FUNCTION_BLOCK IC_KP2_2HB21_IUH_MF
VAR_INPUT
	pADR_IN:								PVOID;					(* Pointer array input data *)
	cbSIZE_IN:								UDINT;					(* Size array input data *)
	pADR_OUT:								PVOID;					(* Pointer array output data *)
	cbSIZE_OUT:								UDINT;					(* Size array output data *)	
	I_T_Timeout : 							TIME;					// Timeout to check command responses
	I_b_StartRead : 						BOOL;					// Trigger to start read command
	I_b_StartWrite : 						BOOL;					// Trigger to start write command
	I_b_StartSpecialCommand : 				BOOL;					// Trigger to start special command (user defined command)
	I_b_UserMemory_UID : 					BOOL;					//0 := access to User Memory; 1 := access to UID/Fixcode
	I_b_EPC : 								BOOL;					//0 := configuration done by Head1UserMemoryUID active; 1 := access to UII/EPC Code (UHF only)
	I_b_SingleEnhanced : 					BOOL;					// 0 = Single command (one-time) ; 1 = Enhanced command (permanent)
	I_b_Quit : 								BOOL;					// Trigger to start Quit command (abort Enhanced command)
	I_w_StartAddress : 						WORD;					// Startaddress of memory access 
	I_i_WordNumber : 						INT;					// Number of blocks
	I_w_TagType : 							WORD;					// TagType
	I_b_WriteParameter : 					BOOL;					//0 := read access to parameter; 1 := write access to parameter
END_VAR
VAR_OUTPUT
	O_b_Done : 								BOOL;					//0 = tag leave detection zone (Enhanced); 1 = tag access successfully executed
	O_b_NoDataCarrier : 					BOOL;					//0 = tag inside/enter detection zone; 1 = no tag or tag leave detection zone
	O_b_Busy : 								BOOL;					//0 = no command actiive; 1 = command active
	O_b_Finish : 							BOOL;					//0 = command active; 1 = command finished
	O_b_Error : 							BOOL;					//0 = no error state; 1 = error state active; check status value
	O_B_Status : 							BYTE;					//Status value of the command response; error information
	O_B_ReplyCounter : 						BYTE;					//Counter of the command responses; increment each new response
	O_b_EndConfig : 						BOOL;					//1 = parameter access finished
END_VAR
VAR_IN_OUT
	IO_b_SetRestart : 						BOOL;					//Trigger initialisation routine
	IO_b_InitFinish : 						BOOL;					//Initialisation routine finished
	IO_b_NewData :							BOOL;					//1 = new data inside data block aviable; direct reset by the user neccessary
	IO_b_StartConfig : 						BOOL;					//1 = trigger of parameter access
	UserDataGlobal 	: 						IDENTControl_UserData_IUH_MF;	//Data block for read/write data and parameter data
END_VAR
VAR
	IDENTControl_FB_MF		: 				IDENTControl_MF;		//Definition of internal function block for Single Frame Protocol
	SpecialCommand_Internal: 				BOOL;					//internal signal for trigger of Special command
	ConfigActive : 							BOOL;					//execution of Special command active
	StateConfig : 							INT;					//state of the execution list
	Done_Internal : 						BOOL;					//Special command finished
	i : 									INT := 0;				//counter
END_VAR

	(*
	#############################################################################################
	
	General Header
	------------------------------------------------------------------------------------------
	Short description:  Function Block for IC-KP2-2HB21 MultiFrame with Parameter configuration for IUH-F19x-V1-FRx-XX
	Version:            1.0
	Name:               IC-KP2-2HB21 Multiframe Protocol with UHF Parameter configuration for IUH-F19x-V1-FRx-XX
	Date:               2024-11-13
	Company:            Pepperl+Fuchs SE
	Author:             Karsten Reinhardt
	EMail:              kreinhardt@de.pepperl-fuchs.com
	Phone:              +49 (0) 621 776 1736

	Changes 1.0: first release
	    - function block include a further function block for standard read/write command without automatic parameter
	    configuration;    
	    - read and write access for different UHF parameter
	
	------------------------------------------------------------------------------------------
	    
	#############################################################################################
	*)

	(*input SpecialCommand hand over to internal signal*)
	SpecialCommand_Internal                   			:= I_b_StartSpecialCommand;

	(*Increase the state of the configuration counter*)
	IF ConfigActive = TRUE AND O_b_Done = TRUE THEN
	    ConfigActive                         			:= FALSE;
	    StateConfig                          			:= StateConfig + 1;
	END_IF;
	
	(*Set Status of the configuration counter to 1 with the trigger for the start of the configuration*)
	IF IO_b_StartConfig = TRUE THEN
	    StateConfig                          			:= 1;
	    IO_b_StartConfig                          		:= FALSE;
	    O_b_EndConfig                             		:= FALSE;
	END_IF;

	IF NOT ConfigActive THEN
	    CASE StateConfig OF
	            
	        0: (* ***** Idle state ***** *)
	            ;
	            
	        1:  (*Additional Information - Parameter IF; transmit a further information telegram with RSSI value;
	            if this parameter is activated a further status 16#0B telegram will transmitted by the evaluation
	            unit; this telegram follows directly after the status 16#00 telegram which contains the read in data
	            of a tag; the status 16#0B telegram with the information will send only one time after the tag is detected;
	            in default setting the parameter is switched off and no additional information are transmit*)
	            IF I_b_WriteParameter = TRUE THEN
	                UserDataGlobal.SpecialCommand[0] 	:= 16#BF;
	            ELSE
					UserDataGlobal.SpecialCommand[0] 	:= 16#BE;	                
	            END_IF;
	            UserDataGlobal.SpecialCommand[1]        := 16#00;
	            UserDataGlobal.SpecialCommand[2]        := 16#00;
	            UserDataGlobal.SpecialCommand[3]        := 16#55;      //SystemCode U
	            UserDataGlobal.SpecialCommand[4]        := 16#49;      //Parameter sign High Byte 'I'
	            UserDataGlobal.SpecialCommand[5]        := 16#46;      //Parameter sign Low Byte 'F'
				IF I_b_WriteParameter = TRUE THEN
	                UserDataGlobal.SpecialCommand[6]    := 16#00;    //Length Parameter High Byte 
	                UserDataGlobal.SpecialCommand[7]    := 16#01;    //Length Parameter Low Byte 
	                UserDataGlobal.SpecialCommand[8]    := UserDataGlobal.WriteParam_IF;    //Parameter value; 16#00 Switched off; 16#01 Switched on
	            ELSE
	                UserDataGlobal.SpecialCommand[6]    := 16#00;    //Length Parameter High Byte 
	                UserDataGlobal.SpecialCommand[7]    := 16#00;    //Length Parameter Low Byte 
	                UserDataGlobal.SpecialCommand[8]    := 16#00;
	            END_IF;
	            SpecialCommand_Internal       			:= TRUE;
	            ConfigActive                 			:= TRUE;            
				
	        2:  (*Antenna Polarisation - Parameter AP; change the polarisation plane of the antenna;
            	in default setting the combined mode is activated. In this case the antenna executes an invetury
            	in horizontal and vertical polarisation plane; this has the advantage that the orientation of the
            	tag can different; of the tag orientation is always identical it is possible to switch to horizontal
            	or vertical polarisation plane; this reduce the execution time for a command*)
	            IF I_b_WriteParameter = TRUE THEN
	                UserDataGlobal.SpecialCommand[0]    := 16#BF;
	            ELSE
	                UserDataGlobal.SpecialCommand[0]    := 16#BE;
	            END_IF;
	            UserDataGlobal.SpecialCommand[1]        := 16#00;
	            UserDataGlobal.SpecialCommand[2]        := 16#00;
	            UserDataGlobal.SpecialCommand[3]        := 16#55;      //SystemCode U
	            UserDataGlobal.SpecialCommand[4]        := 16#41;      //Parameter sign High Byte 'A'
	            UserDataGlobal.SpecialCommand[5]        := 16#50;      //Parameter sign Low Byte 'P'
	            IF I_b_WriteParameter = TRUE THEN
	                UserDataGlobal.SpecialCommand[6]    := 16#00;    //Length Parameter High Byte 
	                UserDataGlobal.SpecialCommand[7]    := 16#01;    //Length Parameter Low Byte 
	                UserDataGlobal.SpecialCommand[8]    := UserDataGlobal.WriteParam_AP;    //Parameter value; 16#43 = Combined Mode; 16#48 = horizontal; 16#56 = vertical
	            ELSE
	                UserDataGlobal.SpecialCommand[6]    := 16#00;    //Length Parameter High Byte 
	                UserDataGlobal.SpecialCommand[7]    := 16#00;    //Length Parameter Low Byte 
	                UserDataGlobal.SpecialCommand[8]    := 16#00;    //Parameter value; 
	            END_IF;
	            SpecialCommand_Internal       			:= TRUE;
	            ConfigActive 							:= TRUE;

	        3:  (*Sending Channels - Parameter CD; used channels on the air interface
            	the FR1-01 devce version uses up to 4 channels on the air interface; with this parameter you can reduce
            	the number of the channels and also define the order of the channels; by reducing the number of channels
            	you achieve a reduction of the execution time; if severla readers are close to each other you can define
            	different air interface channels for the reader to avoid influences*)
	            IF I_b_WriteParameter = TRUE THEN
	                UserDataGlobal.SpecialCommand[0]    := 16#BF;
	            ELSE
	                UserDataGlobal.SpecialCommand[0]    := 16#BE;
	            END_IF;
	            UserDataGlobal.SpecialCommand[1]        := 16#00;
	            UserDataGlobal.SpecialCommand[2]        := 16#00;
	            UserDataGlobal.SpecialCommand[3]        := 16#55;      //SystemCode U
	            UserDataGlobal.SpecialCommand[4]        := 16#43;      //Parameter sign High Byte 'C'
	            UserDataGlobal.SpecialCommand[5]        := 16#44;      //Parameter sign Low Byte 'D'
	            IF I_b_WriteParameter = TRUE THEN
	                UserDataGlobal.SpecialCommand[6]    := INT_TO_BYTE (SHR (UserDataGlobal.Length_CD, 8));    //Length Parameter High Byte 
	                UserDataGlobal.SpecialCommand[7]    := INT_TO_BYTE (UserDataGlobal.Length_CD);    //Length Parameter Low Byte
	                UserDataGlobal.SpecialCommand[8]    := UserDataGlobal.WriteParam_CD[0];    //Parameter value; value Parameter CD
	                UserDataGlobal.SpecialCommand[9]    := UserDataGlobal.WriteParam_CD[1];    //Parameter value; value Parameter CD
	                UserDataGlobal.SpecialCommand[10]   := UserDataGlobal.WriteParam_CD[2];    //Parameter value; value Parameter CD
	                UserDataGlobal.SpecialCommand[11]   := UserDataGlobal.WriteParam_CD[3];    //Parameter value; value Parameter CD
	            ELSE
	                UserDataGlobal.SpecialCommand[6]    := 16#00;    //Length Parameter High Byte 
	                UserDataGlobal.SpecialCommand[7]    := 16#00;    //Length Parameter Low Byte 
	                UserDataGlobal.SpecialCommand[8]    := 16#00;    //Parameter value; 
	                UserDataGlobal.SpecialCommand[9]    := 16#00;    //Parameter value; 
	                UserDataGlobal.SpecialCommand[10]   := 16#00;    //Parameter value; 
	                UserDataGlobal.SpecialCommand[11]   := 16#00;    //Parameter value; 
	            END_IF;
	            SpecialCommand_Internal       			:= TRUE;
	            ConfigActive                 			:= TRUE;			
				
 			4:  (*Enhanced Status 5 - Parameter E5; delay the sending of a status 16#05 telegram which signalise that
            	a tag leaves the detection zone; if there is a inhomogeneous reading zone you have areas in which a tag
           		could not identified; in this case the reader generates a status 16#05 telegram that signalize that a tag 
            	could not accessed; these parameter can delay such telegrams that you can avoid a lot of status 16#05 (no read) 
            	telegrams in a inhomogeneous reading zone*)
	            IF I_b_WriteParameter = TRUE THEN
	                UserDataGlobal.SpecialCommand[0]    := 16#BF;
	            ELSE
	                UserDataGlobal.SpecialCommand[0]    := 16#BE;
	            END_IF;
	            UserDataGlobal.SpecialCommand[1]        := 16#00;
	            UserDataGlobal.SpecialCommand[2]        := 16#00;
	            UserDataGlobal.SpecialCommand[3]        := 16#55;      //SystemCode U
	            UserDataGlobal.SpecialCommand[4]        := 16#45;      //Parameter sign High Byte 'E'
	            UserDataGlobal.SpecialCommand[5]        := 16#35;      //Parameter sign Low Byte '5'
	            IF I_b_WriteParameter = TRUE THEN
	                UserDataGlobal.SpecialCommand[6]    := 16#00;    //Length Parameter High Byte 
	                UserDataGlobal.SpecialCommand[7]    := 16#01;    //Length Parameter Low Byte 
	                UserDataGlobal.SpecialCommand[8]    := UserDataGlobal.WriteParam_E5;    //Parameter value; 16#05 = Default setting
	            ELSE
	                UserDataGlobal.SpecialCommand[6]    := 16#00;    //Length Parameter High Byte 
	                UserDataGlobal.SpecialCommand[7]    := 16#00;    //Length Parameter Low Byte 
	                UserDataGlobal.SpecialCommand[8]    := 16#00;    //Parameter value;
	            END_IF;
	            SpecialCommand_Internal       			:= TRUE;
	            ConfigActive                 			:= TRUE;			
				
	        5: (*Memory Bank - Parameter MB; define to which memory bank the Single/Enhanced Read/Write Words commands
            	get access; in default setting the Read/Write Words command get access to memory bank 16#03 "User Memory";
            	16#00 --> Password Area; 16#01 --> UII/EPC; 16#02 --> TID; 16#03 --> User Memory*)
	            IF I_b_WriteParameter = TRUE THEN
	                UserDataGlobal.SpecialCommand[0]    := 16#BF;
	            ELSE
	                UserDataGlobal.SpecialCommand[0]    := 16#BE;
	            END_IF;
	            UserDataGlobal.SpecialCommand[1]        := 16#00;
	            UserDataGlobal.SpecialCommand[2]        := 16#00;
	            UserDataGlobal.SpecialCommand[3]        := 16#55;      //SystemCode U
	            UserDataGlobal.SpecialCommand[4]        := 16#4D;      //Parameter sign High Byte 'M'
	            UserDataGlobal.SpecialCommand[5]        := 16#42;      //Parameter sign Low Byte 'B'
	            IF I_b_WriteParameter = TRUE THEN
	                UserDataGlobal.SpecialCommand[6]    := 16#00;    //Length Parameter High Byte 
	                UserDataGlobal.SpecialCommand[7]    := 16#01;    //Length Parameter Low Byte 
	                UserDataGlobal.SpecialCommand[8]    := UserDataGlobal.WriteParam_MB;    //Parameter value; Default = 16#03 = User Memory
	            ELSE
	                UserDataGlobal.SpecialCommand[6]    := 16#00;    //Length Parameter High Byte 
	                UserDataGlobal.SpecialCommand[7]    := 16#00;    //Length Parameter Low Byte 
	                UserDataGlobal.SpecialCommand[8]    := 16#00;    //Parameter value; 
	            END_IF;
	            SpecialCommand_Internal       			:= TRUE;
	            ConfigActive                 			:= TRUE;	            	
				
	        6:  (*Number of Tags - Parameter NT; stop criteria to abort the execution of a Single command; this parameter
            	allows the stop of the command execution if one or a defined number of tags are detected; in default setting
            	the parameter has the value 16#FF and the command does not stop before all invetury rounds are executed; if
            	the value 16#01 is defined the command execution of a Single command stops if one tag is detected during an
            	invetury round; if two tags are detected during an inventury round both tags will transmit*)
	            IF I_b_WriteParameter = TRUE THEN
	                UserDataGlobal.SpecialCommand[0]    := 16#BF;
	            ELSE
	                UserDataGlobal.SpecialCommand[0]    := 16#BE;
	            END_IF;
	            UserDataGlobal.SpecialCommand[1]        := 16#00;
	            UserDataGlobal.SpecialCommand[2]        := 16#00;
	            UserDataGlobal.SpecialCommand[3]        := 16#55;      //SystemCode U
	            UserDataGlobal.SpecialCommand[4]        := 16#4E;      //Parameter sign High Byte 'N'
	            UserDataGlobal.SpecialCommand[5]        := 16#54;      //Parameter sign Low Byte 'T'
	            IF I_b_WriteParameter = TRUE THEN
	                UserDataGlobal.SpecialCommand[6]    := 16#00;    //Length Parameter High Byte 
	                UserDataGlobal.SpecialCommand[7]    := 16#01;    //Length Parameter Low Byte 
	                UserDataGlobal.SpecialCommand[8]    := UserDataGlobal.WriteParam_NT;    //Parameter value; Default = 16#FF
	            ELSE
	                UserDataGlobal.SpecialCommand[6]    := 16#00;    //Length Parameter High Byte 
	                UserDataGlobal.SpecialCommand[7]    := 16#00;    //Length Parameter Low Byte 
	                UserDataGlobal.SpecialCommand[8]    := 16#00;    //Parameter value; 
	            END_IF;
	            SpecialCommand_Internal       			:= TRUE;
	            ConfigActive                 			:= TRUE;
	            
	        7:  (*Protocol Mode - Parameter QV; defines the communication protocol of the head; in default setting the
            	head communicates with the MultiFrame protocol; this allows the identification of several tags inside
            	the detection zone; it is possible to switch the protocol to SingleFrame, but than the function block
            	is incompatible*)
	            IF I_b_WriteParameter = TRUE THEN
	                UserDataGlobal.SpecialCommand[0]    := 16#BF;
	            ELSE
	                UserDataGlobal.SpecialCommand[0]    := 16#BE;
	            END_IF;
	            UserDataGlobal.SpecialCommand[1]        := 16#00;
	            UserDataGlobal.SpecialCommand[2]        := 16#00;
	            UserDataGlobal.SpecialCommand[3]        := 16#55;      //SystemCode U
	            UserDataGlobal.SpecialCommand[4]        := 16#51;      //Parameter sign High Byte 'Q'
	            UserDataGlobal.SpecialCommand[5]        := 16#56;      //Parameter sign Low Byte 'V'
	            IF I_b_WriteParameter = TRUE THEN
	                UserDataGlobal.SpecialCommand[6]    := 16#00;    //Length Parameter High Byte 
	                UserDataGlobal.SpecialCommand[7]    := 16#01;    //Length Parameter Low Byte 
	                UserDataGlobal.SpecialCommand[8]    := UserDataGlobal.WriteParam_QV;    //Parameter value; 
	            ELSE
	                UserDataGlobal.SpecialCommand[6]    := 16#00;    //Length Parameter High Byte 
	                UserDataGlobal.SpecialCommand[7]    := 16#00;    //Length Parameter Low Byte 
	                UserDataGlobal.SpecialCommand[8]    := 16#00;    //Parameter value; 
	            END_IF;
	            SpecialCommand_Internal       			:= TRUE;
	            ConfigActive                 			:= TRUE;								

			8:  (*Q Value - Parameter QW; defines the number of time slots on the air interface with 2^Q; the number of
            	time slots should be fit to the number of tags which should be identified*)
	            IF I_b_WriteParameter = TRUE THEN
	                UserDataGlobal.SpecialCommand[0]    := 16#BF;
	            ELSE
	                UserDataGlobal.SpecialCommand[0]    := 16#BE;
	            END_IF;
	            UserDataGlobal.SpecialCommand[1]        := 16#00;
	            UserDataGlobal.SpecialCommand[2]        := 16#00;
	            UserDataGlobal.SpecialCommand[3]        := 16#55;      //SystemCode U
	            UserDataGlobal.SpecialCommand[4]        := 16#51;      //Parameter sign High Byte 'Q'
	            UserDataGlobal.SpecialCommand[5]        := 16#57;      //Parameter sign Low Byte 'W'
	            IF I_b_WriteParameter = TRUE THEN
	                UserDataGlobal.SpecialCommand[6]    := 16#00;    //Length Parameter High Byte 
	                UserDataGlobal.SpecialCommand[7]    := 16#01;    //Length Parameter Low Byte 
	                UserDataGlobal.SpecialCommand[8]    := UserDataGlobal.WriteParam_QW;
	                UserDataGlobal.SpecialCommand[9]    := 16#00;
	            ELSE
	                UserDataGlobal.SpecialCommand[6]    := 16#00;    //Length Parameter High Byte 
	                UserDataGlobal.SpecialCommand[7]    := 16#00;    //Length Parameter Low Byte 
	                UserDataGlobal.SpecialCommand[8]    := 16#00;    //Parameter value; 
	                UserDataGlobal.SpecialCommand[9]    := 16#00;    //Parameter value; 
	            END_IF;
	            SpecialCommand_Internal       			:= TRUE;
	            ConfigActive                 			:= TRUE;	
								
			9:  (*Sensing Mode - Parameter SM; defines a pause time during the execution of Enhanced commands; by increasing
            	the pause time it is possible to reduce the internal heating of the head *)
	            IF I_b_WriteParameter = TRUE THEN
	                UserDataGlobal.SpecialCommand[0]    := 16#BF;
	            ELSE
	                UserDataGlobal.SpecialCommand[0]    := 16#BE;
	            END_IF;
	            UserDataGlobal.SpecialCommand[1]        := 16#00;
	            UserDataGlobal.SpecialCommand[2]        := 16#00;
	            UserDataGlobal.SpecialCommand[3]        := 16#55;      //SystemCode U
	            UserDataGlobal.SpecialCommand[4]        := 16#53;      //Parameter sign High Byte 'S'
	            UserDataGlobal.SpecialCommand[5]        := 16#4D;      //Parameter sign Low Byte 'M'
	            IF I_b_WriteParameter = TRUE THEN
	                UserDataGlobal.SpecialCommand[6]    := 16#00;    //Length Parameter High Byte 
	                UserDataGlobal.SpecialCommand[7]    := 16#02;    //Length Parameter Low Byte 
	                UserDataGlobal.SpecialCommand[8]    := WORD_TO_BYTE (SHR (UserDataGlobal.WriteParam_SM, 8));
					UserDataGlobal.SpecialCommand[9]    := WORD_TO_BYTE (UserDataGlobal.WriteParam_SM);    //Parameter value; 
	            ELSE
	                UserDataGlobal.SpecialCommand[6]    := 16#00;    //Length Parameter High Byte 
	                UserDataGlobal.SpecialCommand[7]    := 16#00;    //Length Parameter Low Byte 
	                UserDataGlobal.SpecialCommand[8]    := 16#00;    //Parameter value; 
	                UserDataGlobal.SpecialCommand[9]    := 16#00;    //Parameter value; 
	            END_IF;
	            SpecialCommand_Internal       			:= TRUE;
	            ConfigActive                 			:= TRUE;							
				
	        10:  (*Tries allowed - Parameter TA; defines the number of allowed tries for the identification of a tag*)
	            IF I_b_WriteParameter = TRUE THEN
	                UserDataGlobal.SpecialCommand[0]    := 16#BF;
	            ELSE
	                UserDataGlobal.SpecialCommand[0]    := 16#BE;
	            END_IF;
	            UserDataGlobal.SpecialCommand[1]        := 16#00;
	            UserDataGlobal.SpecialCommand[2]        := 16#00;
	            UserDataGlobal.SpecialCommand[3]        := 16#55;      //SystemCode U
	            UserDataGlobal.SpecialCommand[4]        := 16#54;      //Parameter sign High Byte 'T'
	            UserDataGlobal.SpecialCommand[5]        := 16#41;      //Parameter sign Low Byte 'A'
	            IF I_b_WriteParameter = TRUE THEN
	                UserDataGlobal.SpecialCommand[6]    := 16#00;    //Length Parameter High Byte 
	                UserDataGlobal.SpecialCommand[7]    := 16#01;    //Length Parameter Low Byte 
	                UserDataGlobal.SpecialCommand[8]    := UserDataGlobal.WriteParam_TA;
	                UserDataGlobal.SpecialCommand[9]    := 16#00;	           
 				ELSE
	                UserDataGlobal.SpecialCommand[6]    := 16#00;    //Length Parameter High Byte 
	                UserDataGlobal.SpecialCommand[7]    := 16#00;    //Length Parameter Low Byte 
	                UserDataGlobal.SpecialCommand[8]    := 16#00;    //Parameter value; 
	            END_IF;
	            SpecialCommand_Internal       			:= TRUE;
	            ConfigActive                 			:= TRUE;				
												
	        11:  (*Power Transmit - Parameter PT; defines the output power of the RFID antenna; it is allowed to define up
            	10 different levels for this parameter; in this case it is possible to generate a ramp for the output power;
           		following levels are possible (in mW) 3, 4, 5, 6, 8, 10, 13, 15, 20, 25, 30, 40, 50, 60, 80, 100, 125, 150,
            	200, 250, 300, 400, 500, 600, 800, 1000, 1250, 1500, 2000*)
	            IF I_b_WriteParameter = TRUE THEN
	                UserDataGlobal.SpecialCommand[0]    := 16#BF;
	            ELSE
	                UserDataGlobal.SpecialCommand[0]    := 16#BE;
	            END_IF;
	            UserDataGlobal.SpecialCommand[1]        := 16#00;
	            UserDataGlobal.SpecialCommand[2]        := 16#00;
	            UserDataGlobal.SpecialCommand[3]        := 16#55;      //SystemCode U
	            UserDataGlobal.SpecialCommand[4]        := 16#50;      //Parameter sign High Byte 'P'
	            UserDataGlobal.SpecialCommand[5]        := 16#54;      //Parameter sign Low Byte 'T'
	            IF I_b_WriteParameter = TRUE THEN
	                UserDataGlobal.SpecialCommand[6]    := INT_TO_BYTE (SHR (UserDataGlobal.Length_PT, 8));    //Length Parameter High Byte 
	                UserDataGlobal.SpecialCommand[7]    := INT_TO_BYTE (UserDataGlobal.Length_PT);    //Length Parameter Low Byte 
	            	UserDataGlobal.SpecialCommand[8]    := WORD_TO_BYTE (SHR (UserDataGlobal.WriteParam_PT[1], 8));
					UserDataGlobal.SpecialCommand[9]	:= WORD_TO_BYTE (UserDataGlobal.WriteParam_PT[1]);
					UserDataGlobal.SpecialCommand[10]   := WORD_TO_BYTE (SHR (UserDataGlobal.WriteParam_PT[2], 8));
					UserDataGlobal.SpecialCommand[11]	:= WORD_TO_BYTE (UserDataGlobal.WriteParam_PT[2]);
					UserDataGlobal.SpecialCommand[12]   := WORD_TO_BYTE (SHR (UserDataGlobal.WriteParam_PT[3], 8));
					UserDataGlobal.SpecialCommand[13]	:= WORD_TO_BYTE (UserDataGlobal.WriteParam_PT[3]);
					UserDataGlobal.SpecialCommand[14]   := WORD_TO_BYTE (SHR (UserDataGlobal.WriteParam_PT[4], 8));
					UserDataGlobal.SpecialCommand[15]	:= WORD_TO_BYTE (UserDataGlobal.WriteParam_PT[4]);
					UserDataGlobal.SpecialCommand[16]   := WORD_TO_BYTE (SHR (UserDataGlobal.WriteParam_PT[5], 8));
					UserDataGlobal.SpecialCommand[17]	:= WORD_TO_BYTE (UserDataGlobal.WriteParam_PT[5]);
					UserDataGlobal.SpecialCommand[18]   := WORD_TO_BYTE (SHR (UserDataGlobal.WriteParam_PT[6], 8));
					UserDataGlobal.SpecialCommand[19]	:= WORD_TO_BYTE (UserDataGlobal.WriteParam_PT[6]);
					UserDataGlobal.SpecialCommand[20]   := WORD_TO_BYTE (SHR (UserDataGlobal.WriteParam_PT[7], 8));
					UserDataGlobal.SpecialCommand[21]	:= WORD_TO_BYTE (UserDataGlobal.WriteParam_PT[7]);
					UserDataGlobal.SpecialCommand[22]   := WORD_TO_BYTE (SHR (UserDataGlobal.WriteParam_PT[8], 8));
					UserDataGlobal.SpecialCommand[23]	:= WORD_TO_BYTE (UserDataGlobal.WriteParam_PT[8]);
					UserDataGlobal.SpecialCommand[24]   := WORD_TO_BYTE (SHR (UserDataGlobal.WriteParam_PT[9], 8));
					UserDataGlobal.SpecialCommand[25]	:= WORD_TO_BYTE (UserDataGlobal.WriteParam_PT[9]);
					UserDataGlobal.SpecialCommand[26]   := WORD_TO_BYTE (SHR (UserDataGlobal.WriteParam_PT[10], 8));
					UserDataGlobal.SpecialCommand[27]	:= WORD_TO_BYTE (UserDataGlobal.WriteParam_PT[10]);
				ELSE
	                UserDataGlobal.SpecialCommand[6]    := 16#00;    //Length Parameter High Byte 
	                UserDataGlobal.SpecialCommand[7]    := 16#00;    //Length Parameter Low Byte 
	                UserDataGlobal.SpecialCommand[8]    := 16#00;    //Parameter value; 
	                UserDataGlobal.SpecialCommand[9]    := 16#00;    //Parameter value; 
	            END_IF;
	            SpecialCommand_Internal 				:= TRUE;
	            ConfigActive 							:= TRUE;
		
				
	        12:    (*Measured Reflection - Parameter MF; read out measured reflection; the measurement of the reflection
                is only possible if the antenna polarisation is horizontal (H) or vertical (V); in default setting
                the parameter AP "antenna polarisation" is defined as "C" combined; in this case the measurement
                is not possible and gives back a status 16#04 error response*)
	            UserDataGlobal.SpecialCommand[0]        := 16#BE;
	            UserDataGlobal.SpecialCommand[1]        := 16#00;
	            UserDataGlobal.SpecialCommand[2]        := 16#00;
	            UserDataGlobal.SpecialCommand[3]        := 16#55;      //SystemCode U
	            UserDataGlobal.SpecialCommand[4]        := 16#4D;      //Parameter sign High Byte 'M'
	            UserDataGlobal.SpecialCommand[5]        := 16#46;      //Parameter sign Low Byte 'F'
	            UserDataGlobal.SpecialCommand[6]        := 16#00;    //Length Parameter High Byte 
	            UserDataGlobal.SpecialCommand[7]        := 16#00;    //Length Parameter Low Byte 
	            UserDataGlobal.SpecialCommand[8]        := 16#00;    //Parameter value; 
	            
	            SpecialCommand_Internal       			:= TRUE;
	            ConfigActive                 			:= TRUE;				
														
	        13: (*Region Code - Parameter RC; defines the region code of the UHF head; by using devices IUH-F190 the
            	region code is only redable because it is predefined and fixed; by using devices IUH-F192 it is neccessary
            	to configure the region code with the first start up; the default setting of the RC by using the IUH-F192
            	is 16#0000; the country specific values you find in the manual of the RFID head*)
	            IF I_b_WriteParameter = TRUE THEN
	                UserDataGlobal.SpecialCommand[0]    := 16#BF;
	            ELSE
	                UserDataGlobal.SpecialCommand[0]    := 16#BE;
	            END_IF;
	            UserDataGlobal.SpecialCommand[1]        := 16#00;
	            UserDataGlobal.SpecialCommand[2]        := 16#00;
	            UserDataGlobal.SpecialCommand[3]        := 16#55;      //SystemCode U
	            UserDataGlobal.SpecialCommand[4]        := 16#52;      //Parameter sign High Byte 'R'
	            UserDataGlobal.SpecialCommand[5]        := 16#43;      //Parameter sign Low Byte 'C'
	            IF I_b_WriteParameter = TRUE THEN
	                UserDataGlobal.SpecialCommand[6]    := 16#00;    //Length Parameter High Byte 
	                UserDataGlobal.SpecialCommand[7]    := 16#02;    //Length Parameter Low Byte 
	                UserDataGlobal.SpecialCommand[8]    := WORD_TO_BYTE (SHR (UserDataGlobal.WriteParam_RC, 8));
	                UserDataGlobal.SpecialCommand[9]    := WORD_TO_BYTE (UserDataGlobal.WriteParam_RC);	           
 				ELSE
	                UserDataGlobal.SpecialCommand[6]    := 16#00;    //Length Parameter High Byte 
	                UserDataGlobal.SpecialCommand[7]    := 16#00;    //Length Parameter Low Byte 
	                UserDataGlobal.SpecialCommand[8]    := 16#00;    //Parameter value; 
	            END_IF;	            
	            SpecialCommand_Internal       			:= TRUE;
	            ConfigActive                 			:= TRUE;											
				
	        14: (*Number of Channels - Parameter NC; this parameter defines the number of used channels on the air interface;
            	by using heads of the FR1 frequency range this parameter is only readable; by using heads of the FR2 frequency
            	range this parameter can write; possible values you find in the manual of the RFID head *)
	            IF I_b_WriteParameter = TRUE THEN
	                UserDataGlobal.SpecialCommand[0]    := 16#BF;
	            ELSE
	                UserDataGlobal.SpecialCommand[0]    := 16#BE;
	            END_IF;
	            UserDataGlobal.SpecialCommand[1]        := 16#00;
	            UserDataGlobal.SpecialCommand[2]        := 16#00;
	            UserDataGlobal.SpecialCommand[3]        := 16#55;      //SystemCode U
	            UserDataGlobal.SpecialCommand[4]        := 16#4E;      //Parameter sign High Byte 'N'
	            UserDataGlobal.SpecialCommand[5]        := 16#43;      //Parameter sign Low Byte 'C'
	            IF I_b_WriteParameter = TRUE THEN
	                UserDataGlobal.SpecialCommand[6]    := 16#00;    //Length Parameter High Byte 
	                UserDataGlobal.SpecialCommand[7]    := 16#01;    //Length Parameter Low Byte 
	                UserDataGlobal.SpecialCommand[8]    := UserDataGlobal.WriteParam_NC;
	                UserDataGlobal.SpecialCommand[9]    := 16#00;	           
 				ELSE
	                UserDataGlobal.SpecialCommand[6]    := 16#00;    //Length Parameter High Byte 
	                UserDataGlobal.SpecialCommand[7]    := 16#00;    //Length Parameter Low Byte 
	                UserDataGlobal.SpecialCommand[8]    := 16#00;    //Parameter value; 
	            END_IF;
	            
	            SpecialCommand_Internal       			:= TRUE;
	            ConfigActive                 			:= TRUE;								
			
	        15:  (*Filter Mask - Parameter FL; read out Filter Mask 0*)
	            UserDataGlobal.SpecialCommand[0]        := 16#BE;
	            UserDataGlobal.SpecialCommand[1]        := 16#00;
	            UserDataGlobal.SpecialCommand[2]        := 16#00;
	            UserDataGlobal.SpecialCommand[3]        := 16#55;      //SystemCode U
	            UserDataGlobal.SpecialCommand[4]        := 16#46;      //Parameter sign High Byte 'F'
	            UserDataGlobal.SpecialCommand[5]        := 16#4C;      //Parameter sign Low Byte 'L'
	            UserDataGlobal.SpecialCommand[6]        := 16#00;    //Length Parameter High Byte 
	            UserDataGlobal.SpecialCommand[7]        := 16#01;    //Length Parameter Low Byte 
	            UserDataGlobal.SpecialCommand[8]        := 16#00;    //Parameter value; 
	            
	            SpecialCommand_Internal       			:= TRUE;
	            ConfigActive                 			:= TRUE;				
				
			16:  (*Filter Mask - Parameter FL; read out Filter Mask 1*)
	            UserDataGlobal.SpecialCommand[0]        := 16#BE;
	            UserDataGlobal.SpecialCommand[1]        := 16#00;
	            UserDataGlobal.SpecialCommand[2]        := 16#00;
	            UserDataGlobal.SpecialCommand[3]        := 16#55;      //SystemCode U
	            UserDataGlobal.SpecialCommand[4]        := 16#46;      //Parameter sign High Byte 'F'
	            UserDataGlobal.SpecialCommand[5]        := 16#4C;      //Parameter sign Low Byte 'L'
	            UserDataGlobal.SpecialCommand[6]        := 16#00;    //Length Parameter High Byte 
	            UserDataGlobal.SpecialCommand[7]        := 16#01;    //Length Parameter Low Byte 
	            UserDataGlobal.SpecialCommand[8]        := 16#01;    //Parameter value; 
	            
				SpecialCommand_Internal       			:= TRUE;
	            ConfigActive                 			:= TRUE;
														
	        17:  (*Filter Mask - Parameter FL; read out Filter Mask 2*)
	            UserDataGlobal.SpecialCommand[0]        := 16#BE;
	            UserDataGlobal.SpecialCommand[1]        := 16#00;
	            UserDataGlobal.SpecialCommand[2]        := 16#00;
	            UserDataGlobal.SpecialCommand[3]        := 16#55;      //SystemCode U
	            UserDataGlobal.SpecialCommand[4]        := 16#46;      //Parameter sign High Byte 'F'
	            UserDataGlobal.SpecialCommand[5]        := 16#4C;      //Parameter sign Low Byte 'L'
	            UserDataGlobal.SpecialCommand[6]        := 16#00;    //Length Parameter High Byte 
	            UserDataGlobal.SpecialCommand[7]        := 16#01;    //Length Parameter Low Byte 
	            UserDataGlobal.SpecialCommand[8]        := 16#02;    //Parameter value; 
	            
	            SpecialCommand_Internal       			:= TRUE;
	            ConfigActive                 			:= TRUE;				
				
	        18:  (*Session - Parameter SE; defines the used Session configuration for tag access; HIDDEN PARAMETER!!
            	DO NOT CHANGE!! ONLY FOR SERVICE!!*)
	            IF I_b_WriteParameter = TRUE THEN
	                UserDataGlobal.SpecialCommand[0]    := 16#BF;
	            ELSE
	                UserDataGlobal.SpecialCommand[0]    := 16#BE;
	            END_IF;
	            UserDataGlobal.SpecialCommand[1]        := 16#00;
	            UserDataGlobal.SpecialCommand[2]        := 16#00;
	            UserDataGlobal.SpecialCommand[3]        := 16#55;      //SystemCode U
	            UserDataGlobal.SpecialCommand[4]        := 16#53;      //Parameter sign High Byte 'S'
	            UserDataGlobal.SpecialCommand[5]        := 16#45;      //Parameter sign Low Byte 'E'
	            IF I_b_WriteParameter = TRUE THEN
	                UserDataGlobal.SpecialCommand[6]    := 16#00;    //Length Parameter High Byte 
	                UserDataGlobal.SpecialCommand[7]    := 16#01;    //Length Parameter Low Byte 
	                UserDataGlobal.SpecialCommand[8]    := UserDataGlobal.WriteParam_SE;
	                UserDataGlobal.SpecialCommand[9]    := 16#00;	           
 				ELSE
	                UserDataGlobal.SpecialCommand[6]    := 16#00;    //Length Parameter High Byte 
	                UserDataGlobal.SpecialCommand[7]    := 16#00;    //Length Parameter Low Byte 
	                UserDataGlobal.SpecialCommand[8]    := 16#00;    //Parameter value; 
	            END_IF;
	            
	            SpecialCommand_Internal       			:= TRUE;
	            ConfigActive                 			:= TRUE;				
				
	        19:  (*Search Mode - Parameter FB; Defines the search mode of the head; HIDDEN PARAMETER!!
            	DO NOT CHANGE!! ONLY FOR SERVICE!!*)
	            IF I_b_WriteParameter = TRUE THEN
	                UserDataGlobal.SpecialCommand[0]    := 16#BF;
	            ELSE
	                UserDataGlobal.SpecialCommand[0]    := 16#BE;
	            END_IF;
	            UserDataGlobal.SpecialCommand[1]        := 16#00;
	            UserDataGlobal.SpecialCommand[2]        := 16#00;
	            UserDataGlobal.SpecialCommand[3]        := 16#55;      //SystemCode U
	            UserDataGlobal.SpecialCommand[4]        := 16#46;      //Parameter sign High Byte 'F'
	            UserDataGlobal.SpecialCommand[5]        := 16#42;      //Parameter sign Low Byte 'B'
	            IF I_b_WriteParameter = TRUE THEN
	                UserDataGlobal.SpecialCommand[6]    := 16#00;    //Length Parameter High Byte 
	                UserDataGlobal.SpecialCommand[7]    := 16#01;    //Length Parameter Low Byte 
	                UserDataGlobal.SpecialCommand[8]    := UserDataGlobal.WriteParam_FB;
	                UserDataGlobal.SpecialCommand[9]    := 16#00;	           
 				ELSE
	                UserDataGlobal.SpecialCommand[6]    := 16#00;    //Length Parameter High Byte 
	                UserDataGlobal.SpecialCommand[7]    := 16#00;    //Length Parameter Low Byte 
	                UserDataGlobal.SpecialCommand[8]    := 16#00;    //Parameter value; 
	            END_IF;
	            
	            SpecialCommand_Internal       			:= TRUE;
	            ConfigActive                 			:= TRUE;	           
 
	        20: (*First Read - Parameter FR; defines the write access to the tag; HIDDEN PARAMETER!!
            	DO NOT CHANGE!! ONLY FOR SERVICE!!*)
	            IF I_b_WriteParameter = TRUE THEN
	                UserDataGlobal.SpecialCommand[0]    := 16#BF;
	            ELSE
	                UserDataGlobal.SpecialCommand[0]    := 16#BE;
	            END_IF;
	            UserDataGlobal.SpecialCommand[1]        := 16#00;
	            UserDataGlobal.SpecialCommand[2]        := 16#00;
	            UserDataGlobal.SpecialCommand[3]        := 16#55;      //SystemCode U
	            UserDataGlobal.SpecialCommand[4]        := 16#46;      //Parameter sign High Byte 'F'
	            UserDataGlobal.SpecialCommand[5]        := 16#52;      //Parameter sign Low Byte 'R'
	            IF I_b_WriteParameter = TRUE THEN
	                UserDataGlobal.SpecialCommand[6]    := 16#00;    //Length Parameter High Byte 
	                UserDataGlobal.SpecialCommand[7]    := 16#01;    //Length Parameter Low Byte 
	                UserDataGlobal.SpecialCommand[8]    := UserDataGlobal.WriteParam_FR;
	                UserDataGlobal.SpecialCommand[9]    := 16#00;	           
 				ELSE
	                UserDataGlobal.SpecialCommand[6]    := 16#00;    //Length Parameter High Byte 
	                UserDataGlobal.SpecialCommand[7]    := 16#00;    //Length Parameter Low Byte 
	                UserDataGlobal.SpecialCommand[8]    := 16#00;    //Parameter value; 
	            END_IF; 
	            
	            SpecialCommand_Internal 				:= TRUE;
	            ConfigActive 							:= TRUE;				
				
			21: (*Fixcode length - Parameter EF; defines the Fixcode length; HIDDEN PARAMETER!!
            	DO NOT CHANGE!! ONLY FOR SERVICE!!*)
	            IF I_b_WriteParameter = TRUE THEN
	                UserDataGlobal.SpecialCommand[0]    := 16#BF;
	            ELSE
	                UserDataGlobal.SpecialCommand[0]    := 16#BE;
	            END_IF;
	            UserDataGlobal.SpecialCommand[1]        := 16#00;
	            UserDataGlobal.SpecialCommand[2]        := 16#00;
	            UserDataGlobal.SpecialCommand[3]        := 16#55;      //SystemCode U
	            UserDataGlobal.SpecialCommand[4]        := 16#45;      //Parameter sign High Byte 'E'
	            UserDataGlobal.SpecialCommand[5]        := 16#46;      //Parameter sign Low Byte 'F'
	            IF I_b_WriteParameter = TRUE THEN
	                UserDataGlobal.SpecialCommand[6]    := 16#00;    //Length Parameter High Byte 
	                UserDataGlobal.SpecialCommand[7]    := 16#01;    //Length Parameter Low Byte 
	                UserDataGlobal.SpecialCommand[8]    := UserDataGlobal.WriteParam_EF;
	                UserDataGlobal.SpecialCommand[9]    := 16#00;	           
 				ELSE
	                UserDataGlobal.SpecialCommand[6]    := 16#00;    //Length Parameter High Byte 
	                UserDataGlobal.SpecialCommand[7]    := 16#00;    //Length Parameter Low Byte 
	                UserDataGlobal.SpecialCommand[8]    := 16#00;    //Parameter value; 
	            END_IF; 
	            
	            SpecialCommand_Internal 				:= TRUE;
	            ConfigActive 							:= TRUE;
								
	        22:
	            StateConfig                  			:= 0; (* Go to idle state *)
	            
	    END_CASE;
	END_IF;	
	
IDENTControl_FB_MF(
	pADR_IN	:= pADR_IN,									(* Pointer array input data *)
	cbSIZE_IN := cbSIZE_IN,								(* Size array input data *)
	pADR_OUT := pADR_OUT,								(* Pointer array output data *)
	cbSIZE_OUT := cbSIZE_OUT,							(* Size array output data *)
	I_T_Timeout := I_T_Timeout, 						// Timeout to check command responses
	I_b_StartRead := I_b_StartRead, 					// Trigger to start read command
	I_b_StartWrite := I_b_StartWrite, 					// Trigger to start write command
	I_b_StartSpecialCommand	:= SpecialCommand_Internal, // Trigger to start special command (user defined command)
	I_b_UserMemory_UID := I_b_UserMemory_UID, 			//0 := access to User Memory; 1 := access to UID/Fixcode
	I_b_EPC := I_b_EPC,									//0 := configuration done by Head1UserMemoryUID active; 1 := access to UII/EPC Code (UHF only)
	I_b_SingleEnhanced := I_b_SingleEnhanced , 			// 0 = Single command (one-time) ; 1 = Enhanced command (permanent)
	I_b_Quit := I_b_Quit, 								// Trigger to start Quit command (abort Enhanced command)
	I_w_StartAddress := I_w_StartAddress, 				// Startaddress of memory access 
	I_i_WordNumber := I_i_WordNumber,					// Number of blocks 
	I_w_TagType := I_w_TagType, 						// TagType
	O_b_Done => Done_Internal, 							//0 = tag leave detection zone (Enhanced); 1 = tag access successfully executed
	O_b_NoDataCarrier => O_b_NoDataCarrier, 			//0 = tag inside/enter detection zone; 1 = no tag or tag leave detection zone
	O_b_Busy => O_b_Busy, 								//0 = no command actiive; 1 = command active
	O_b_Finish => O_b_Finish, 							//0 = command active; 1 = command finished
	O_b_Error => O_b_Error, 							//0 = no error state; 1 = error state active; check status value
	O_B_Status => O_B_Status, 							//Status value of the command response; error information
	O_B_ReplyCounter => O_B_ReplyCounter,				//Counter of the command responses; increment each new response
	IO_b_SetRestart := IO_b_SetRestart, 				//Trigger initialisation routine
	IO_b_InitFinish := IO_b_InitFinish,					//Initialisation routine finished
	IO_b_NewData := IO_b_NewData,
	UserData := UserDataGlobal							//Data block for read/write data
	);
	
	(*Copy read in information from parameter IF*)
	IF StateConfig = 1 AND Done_Internal = TRUE THEN
	    UserDataGlobal.ReadParam_IF               			:= UserDataGlobal.ReadData[0];
	END_IF;
	(*Copy read in information from parameter AP*)
	IF StateConfig = 2 AND Done_Internal = TRUE THEN
	    UserDataGlobal.ReadParam_AP               			:= UserDataGlobal.ReadData[0];
	END_IF;
	(*Copy read in information from parameter CD*)
	IF StateConfig = 3 AND Done_Internal = TRUE THEN
	    UserDataGlobal.ReadParam_CD[0]               		:= UserDataGlobal.ReadData[0];
		UserDataGlobal.ReadParam_CD[1]               		:= UserDataGlobal.ReadData[1];
		UserDataGlobal.ReadParam_CD[2]               		:= UserDataGlobal.ReadData[2];
		UserDataGlobal.ReadParam_CD[3]               		:= UserDataGlobal.ReadData[3];
	END_IF;
	(*Copy read in information from parameter E5*)
	IF StateConfig = 4 AND Done_Internal = TRUE THEN
	    UserDataGlobal.ReadParam_E5               			:= UserDataGlobal.ReadData[0];
	END_IF;	
	(*Copy read in information from parameter MB*)
	IF StateConfig = 5 AND Done_Internal = TRUE THEN
		UserDataGlobal.ReadParam_MB 						:= UserDataGlobal.ReadData[0];
	END_IF;
	(*Copy read in information from parameter NT*)
	IF StateConfig = 6 AND Done_Internal = TRUE THEN
	    UserDataGlobal.ReadParam_NT               			:= UserDataGlobal.ReadData[0];
	END_IF;
	(*Copy read in information from parameter QV*)
	IF StateConfig = 7 AND Done_Internal = TRUE THEN
	    UserDataGlobal.ReadParam_QV               			:= UserDataGlobal.ReadData[0];
	END_IF;
	(*Copy read in information from parameter PT*)
	IF StateConfig = 8 AND Done_internal = TRUE THEN
	    UserDataGlobal.ReadParam_QW 						:= UserDataGlobal.ReadData[0];
	END_IF;	
	(*Copy read in information from parameter SM*)
	IF StateConfig = 9 AND Done_internal = TRUE THEN
	    UserDataGlobal.ReadParam_SM               			:= SHL (BYTE_TO_WORD(UserDataGlobal.ReadData[0]), 8) OR BYTE_TO_WORD (UserDataGlobal.ReadData[1]);
	END_IF;	
	(*Copy read in information from parameter TA*)
	IF StateConfig = 10 AND Done_internal = TRUE THEN
	    UserDataGlobal.ReadParam_TA 						:= UserDataGlobal.ReadData[0];
	END_IF;
	(*Copy read in information from parameter PT*)
	IF StateConfig = 11 AND Done_internal = TRUE THEN
	    UserDataGlobal.ReadParam_PT[1]               		:= SHL (BYTE_TO_WORD(UserDataGlobal.ReadData[0]), 8) OR BYTE_TO_WORD (UserDataGlobal.ReadData[1]);
		UserDataGlobal.ReadParam_PT[2]               		:= SHL (BYTE_TO_WORD(UserDataGlobal.ReadData[2]), 8) OR BYTE_TO_WORD (UserDataGlobal.ReadData[3]);
		UserDataGlobal.ReadParam_PT[3]               		:= SHL (BYTE_TO_WORD(UserDataGlobal.ReadData[4]), 8) OR BYTE_TO_WORD (UserDataGlobal.ReadData[5]);
		UserDataGlobal.ReadParam_PT[4]               		:= SHL (BYTE_TO_WORD(UserDataGlobal.ReadData[6]), 8) OR BYTE_TO_WORD (UserDataGlobal.ReadData[7]);
		UserDataGlobal.ReadParam_PT[5]               		:= SHL (BYTE_TO_WORD(UserDataGlobal.ReadData[8]), 8) OR BYTE_TO_WORD (UserDataGlobal.ReadData[9]);
	    UserDataGlobal.ReadParam_PT[6]               		:= SHL (BYTE_TO_WORD(UserDataGlobal.ReadData[10]), 8) OR BYTE_TO_WORD (UserDataGlobal.ReadData[11]);
	    UserDataGlobal.ReadParam_PT[7]               		:= SHL (BYTE_TO_WORD(UserDataGlobal.ReadData[12]), 8) OR BYTE_TO_WORD (UserDataGlobal.ReadData[13]);
		UserDataGlobal.ReadParam_PT[8]               		:= SHL (BYTE_TO_WORD(UserDataGlobal.ReadData[14]), 8) OR BYTE_TO_WORD (UserDataGlobal.ReadData[15]);
	    UserDataGlobal.ReadParam_PT[9]               		:= SHL (BYTE_TO_WORD(UserDataGlobal.ReadData[16]), 8) OR BYTE_TO_WORD (UserDataGlobal.ReadData[17]);
	    UserDataGlobal.ReadParam_PT[10]               		:= SHL (BYTE_TO_WORD(UserDataGlobal.ReadData[18]), 8) OR BYTE_TO_WORD (UserDataGlobal.ReadData[19]);
	END_IF;		
	(*Copy read in information from parameter MF*)
	IF StateConfig = 12 AND Done_internal = TRUE THEN
		FOR i := 0 TO 51 BY 1 DO
		UserDataGlobal.ReadParam_MF[i]            			:= UserDataGlobal.ReadData[i];	
		END_FOR;	    
	END_IF;	
	(*Copy read in information from parameter RC*)
	IF StateConfig = 13 AND Done_internal = TRUE THEN
		UserDataGlobal.ReadParam_RC               			:= SHL (BYTE_TO_WORD(UserDataGlobal.ReadData[0]), 8) OR BYTE_TO_WORD (UserDataGlobal.ReadData[1]);
	 END_IF;
	(*Copy read in information from parameter NC*)
	IF StateConfig = 14 AND Done_internal = TRUE THEN
	    UserDataGlobal.ReadParam_NC            				:= UserDataGlobal.ReadData[0];
	END_IF;	
	(*Copy read in information from parameter FL 0*)
	IF StateConfig = 15 AND Done_internal = TRUE THEN
	 	FOR i := 0 TO 19 BY 1 DO
		UserDataGlobal.ReadParam_FL_0[i]            		:= UserDataGlobal.ReadData[i];	
		END_FOR;	    
	END_IF;
	(*Copy read in information from parameter FL 1*)
	IF StateConfig = 16 AND Done_internal = TRUE THEN
	    FOR i := 0 TO 19 BY 1 DO
		UserDataGlobal.ReadParam_FL_1[i]            		:= UserDataGlobal.ReadData[i];	
		END_FOR;
	END_IF;
	(*Copy read in information from parameter FL 2*)
	IF StateConfig = 17 AND Done_internal = TRUE THEN
	    FOR i := 0 TO 19 BY 1 DO
		UserDataGlobal.ReadParam_FL_2[i]            		:= UserDataGlobal.ReadData[i];	
		END_FOR;
	END_IF;
	(*Copy read in information from parameter SE*)
	IF StateConfig = 18 AND Done_internal = TRUE THEN
	    UserDataGlobal.ReadParam_SE            				:= UserDataGlobal.ReadData[0];
	END_IF;	
	(*Copy read in information from parameter FB*)
	IF StateConfig = 19 AND Done_internal = TRUE THEN
	    UserDataGlobal.ReadParam_FB               			:= UserDataGlobal.ReadData[0];
	END_IF;
	(*Copy read in information from parameter ST*)
	IF StateConfig = 20 AND Done_internal = TRUE THEN
	    UserDataGlobal.ReadParam_FR							:= UserDataGlobal.ReadData[0];
	END_IF;		
		(*Copy read in information from parameter ST*)
	IF StateConfig = 21 AND Done_internal = TRUE THEN
	    UserDataGlobal.ReadParam_EF							:= UserDataGlobal.ReadData[0];
	END_IF;	
	IF StateConfig = 21 AND Done_Internal = TRUE THEN
	    O_b_EndConfig 										:= TRUE;
	END_IF;
	
	O_b_Done                                      			:= Done_internal;
	
	IF SpecialCommand_Internal = TRUE THEN
	    SpecialCommand_Internal                  			:= FALSE;
	END_IF;

END_FUNCTION_BLOCK
